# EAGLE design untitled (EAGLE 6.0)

## Sheet 1 of 3: NAP a SERVO
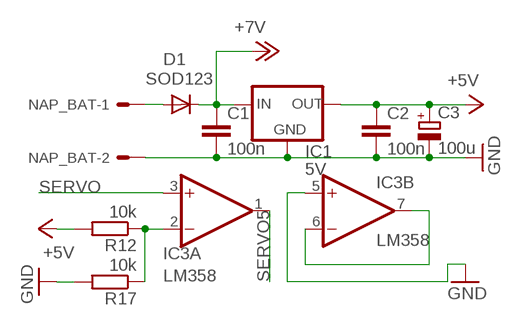
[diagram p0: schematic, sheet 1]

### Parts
C1  100n  C-EUC0805K  [C0805K]
C2  100n  C-EUC0805K  [C0805K]
C3  100u  CPOL-EUE2-5  [E2-5]
D1  SOD123  CGRM4001-G  [SOD-123_MINI-SMA]
IC1  5V  78XXL  [78XXL]
IC3  LM358  TL072D  [SO08]
NAP_BAT  22-27-2021-02  [6410-02]
R12  10k  R-EU_0207/10  [0207/10]
R17  10k  R-EU_0207/10  [0207/10]

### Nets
+7V: C1.1 D1.C IC1.IN ; also sheet 2
GND: C1.2 C2.2 C3.- IC1.GND IC3.5(B:+IN) NAP_BAT.2 R17.2 ; also sheet 2,3
N$2: D1.A NAP_BAT.1
N$6: IC3.6(B:-IN) IC3.7(B:OUT)
N$14: IC3.2(A:-IN) R12.1 R17.1
SERVO: IC3.3(A:+IN) ; also sheet 2
SERVO5: IC3.1(A:OUT) ; also sheet 2
VCC: C2.1 C3.+ IC1.OUT R12.2 ; supply symbol labelled +5V ; also sheet 2,3

## Sheet 2 of 3: HEADER_IO
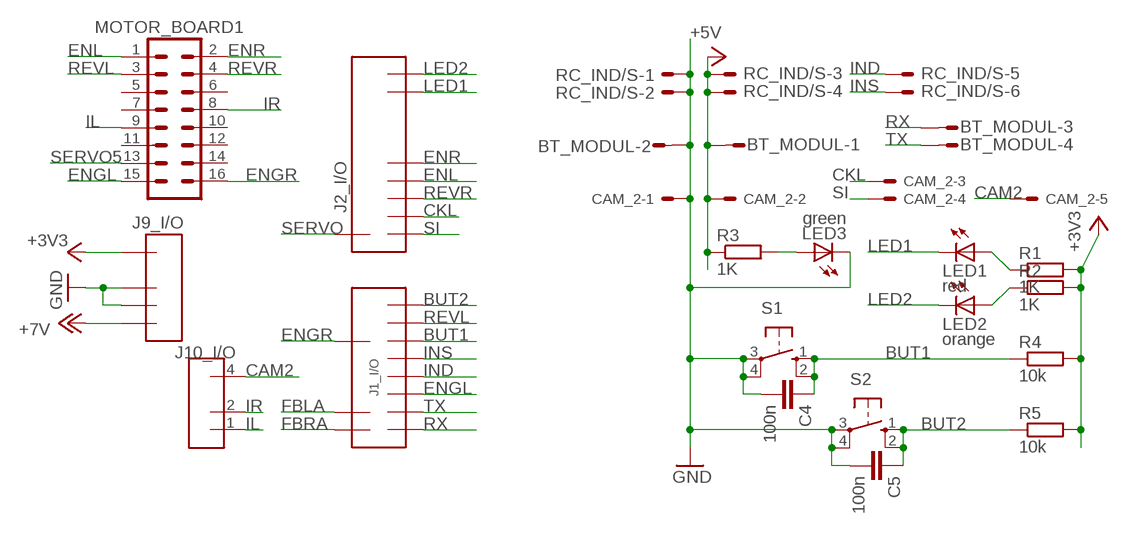
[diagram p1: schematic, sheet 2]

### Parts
BT_MODUL  M04S  [04P]
C4  100n  C-EUC0805K  [C0805K]
C5  100n  C-EUC0805K  [C0805K]
CAM_2  22-27-2051-05  [6410-05]
J1_I/O  DOLNE  [DOLNE]
J2_I/O  HORNE  [HORNE]
J9_I/O  NAP  [NAP]
J10_I/O  ANALOG  [ANALOG]
LED1  red  LED3MM  [LED3MM]
LED2  orange  LED3MM  [LED3MM]
LED3  green  LED3MM  [LED3MM]
MOTOR_BOARD1  ML16  [ML16]
R1  1K  R-EU_R0805  [R0805]
R2  1K  R-EU_R0805  [R0805]
R3  1K  R-EU_R0603  [R0603]
R4  10k  R-EU_R0805  [R0805]
R5  10k  R-EU_R0805  [R0805]
RC_IND/S  ML6E  [ML6]
S1  10-XX  [B3F-10XX]
S2  10-XX  [B3F-10XX]

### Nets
+3V3: J9_I/O.1 R1.2 R2.2 R4.2 R5.2
+7V: J9_I/O.4 ; also sheet 1
BUT1: C4.1 J1_I/O.P$9 R4.1 S1.1(S) S1.2(S1)
BUT2: C5.1 J1_I/O.P$11 R5.1 S2.1(S) S2.2(S1)
CAM2: CAM_2.5 J10_I/O.4
CKL: CAM_2.3 J2_I/O.P$3
ENGL: J1_I/O.P$5 MOTOR_BOARD1.15
ENGR: J1_I/O.P$8 MOTOR_BOARD1.16
ENL: J2_I/O.P$5 MOTOR_BOARD1.1
ENR: J2_I/O.P$6 MOTOR_BOARD1.2
FBLA: J1_I/O.P$3 ; also sheet 3
FBRA: J1_I/O.P$1 ; also sheet 3
GND: BT_MODUL.2 C4.2 C5.2 CAM_2.1 J9_I/O.2 J9_I/O.3 LED3.K(C) RC_IND/S.1 RC_IND/S.2 S1.3(P) S1.4(P1) S2.3(P) S2.4(P1) ; also sheet 1,3
IL: J10_I/O.1 MOTOR_BOARD1.9
IND: J1_I/O.P$6 RC_IND/S.5
INS: J1_I/O.P$7 RC_IND/S.6
IR: J10_I/O.2 MOTOR_BOARD1.8
LED1: J2_I/O.P$7 LED1.K(C)
LED2: J2_I/O.P$8 LED2.K(C)
N$1: LED1.A R1.1
N$15: LED2.A R2.1
N$16: LED3.A R3.2
REVL: J1_I/O.P$10 MOTOR_BOARD1.3
REVR: J2_I/O.P$4 MOTOR_BOARD1.4
RX: BT_MODUL.3 J1_I/O.P$2
SERVO: J2_I/O.P$1 ; also sheet 1
SERVO5: MOTOR_BOARD1.13 ; also sheet 1
SI: CAM_2.4 J2_I/O.P$2
TX: BT_MODUL.4 J1_I/O.P$4
VCC: BT_MODUL.1 CAM_2.2 R3.1 RC_IND/S.3 RC_IND/S.4 ; supply symbol labelled +5V ; also sheet 1,3
Unconnected: MOTOR_BOARD1.5 MOTOR_BOARD1.6 MOTOR_BOARD1.7 MOTOR_BOARD1.10 MOTOR_BOARD1.11 MOTOR_BOARD1.12 MOTOR_BOARD1.14

## Sheet 3 of 3: CNY70
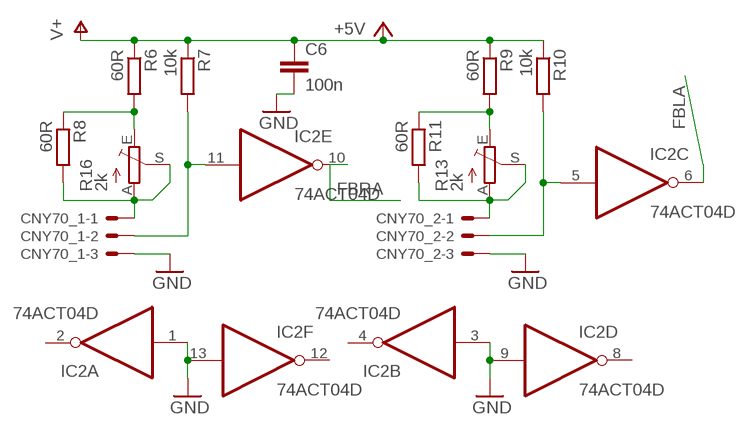
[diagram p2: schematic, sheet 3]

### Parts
C6  100n  C-EUC0805K  [C0805K]
CNY70_1  22-27-2031-03  [6410-03]
CNY70_2  22-27-2031-03  [6410-03]
IC2  74ACT04D  [SO14]
R6  60R  R-EU_R0603  [R0603]
R7  10k  R-EU_R0603  [R0603]
R8  60R  R-EU_R0603  [R0603]
R9  60R  R-EU_R0603  [R0603]
R10  10k  R-EU_R0603  [R0603]
R11  60R  R-EU_R0603  [R0603]
R13  2k  TRIM_EU-CA6V  [CA6V]
R16  2k  TRIM_EU-CA6V  [CA6V]

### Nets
FBLA: IC2.6(C:O) ; also sheet 2
FBRA: IC2.10(E:O) ; also sheet 2
GND: C6.2 CNY70_1.3 CNY70_2.3 IC2.1(A:I) IC2.3(B:I) IC2.9(D:I) IC2.13(F:I) ; also sheet 1,2
N$3: R9.2 R11.1 R13.E
N$4: R6.2 R8.1 R16.E
N$5: CNY70_2.1 R11.2 R13.A R13.S
N$8: CNY70_1.1 R8.2 R16.A R16.S
N$9: CNY70_1.2 IC2.11(E:I) R7.2
N$10: CNY70_2.2 IC2.5(C:I) R10.2
VCC: C6.1 R6.1 R7.1 R9.1 R10.1 ; supply symbol labelled V+, +5V ; also sheet 1,2
Unconnected: IC2.2(A:O) IC2.4(B:O) IC2.8(D:O) IC2.12(F:O)

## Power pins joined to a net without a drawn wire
GND: IC2.7(P:GND) IC3.4(P:V-)
VCC: IC2.14(P:VCC) IC3.8(P:V+)

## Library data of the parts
BT_MODUL = con-amp-quick:M04S: AMP QUICK CONNECTOR; OC_FARNELL: unknown; OC_NEWARK: unknown
C1 C2 C4-C6 = rcl:C-EU: CAPACITOR, European symbol
C3 = rcl:CPOL-EU: POLARIZED CAPACITOR, European symbol
CAM_2 = con-molex:22-?-05: CONNECTOR wire to board 2.54 mm (.1 inch) pitch header; OC_FARNELL: unknown; OC_NEWARK: unknown
CNY70_1 CNY70_2 = con-molex:22-?-03: CONNECTOR wire to board 2.54 mm (.1 inch) pitch header; OC_FARNELL: unknown; OC_NEWARK: unknown
D1 = diode:CGRM400*-G: Molded plasitc,JEDEC SOD-123/Mini SMA
IC1 = v-reg:78XXL: VOLTAGE REGULATOR
IC2 = 74xx-eu:74*04: Hex INVERTER
IC3 = linear:TL072: OP AMP
J1_I/O = con-tfc:DOLNE
J2_I/O = con-tfc:HORNE
J9_I/O = con-tfc:NAP
J10_I/O = con-tfc:ANALOG
LED1-LED3 = led:LED: LED
MOTOR_BOARD1 = con-ml:ML16: HARTING; OC_FARNELL: unknown; OC_NEWARK: unknown
NAP_BAT = con-molex:22-?-02: CONNECTOR; OC_FARNELL: unknown; OC_NEWARK: unknown
R1-R12 R17 = rcl:R-EU_: RESISTOR, European symbol
R13 R16 = pot:TRIM_EU-: POTENTIOMETER
RC_IND/S = con-ml:ML6E: HARTING; OC_FARNELL: unknown; OC_NEWARK: unknown
S1 S2 = switch-omron:10-XX: OMRON SWITCH; MPN: B3F-1000; OC_FARNELL: 176432; OC_NEWARK: 36M3542

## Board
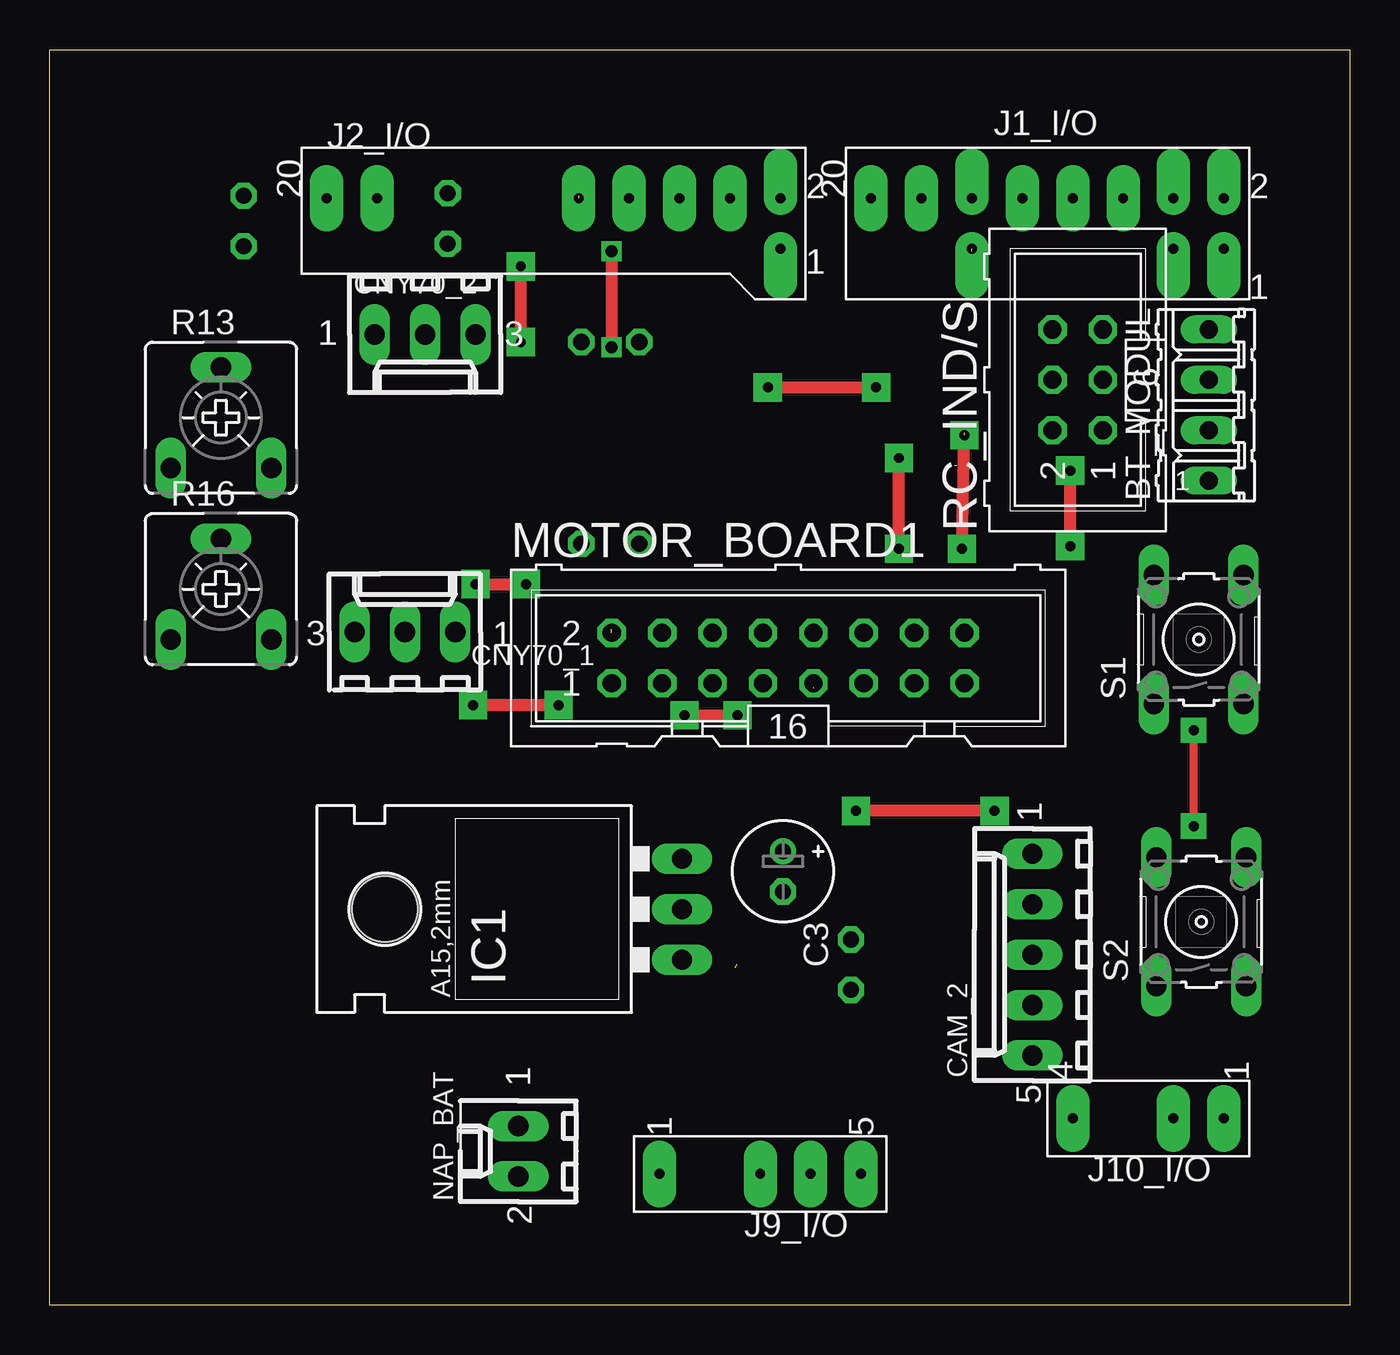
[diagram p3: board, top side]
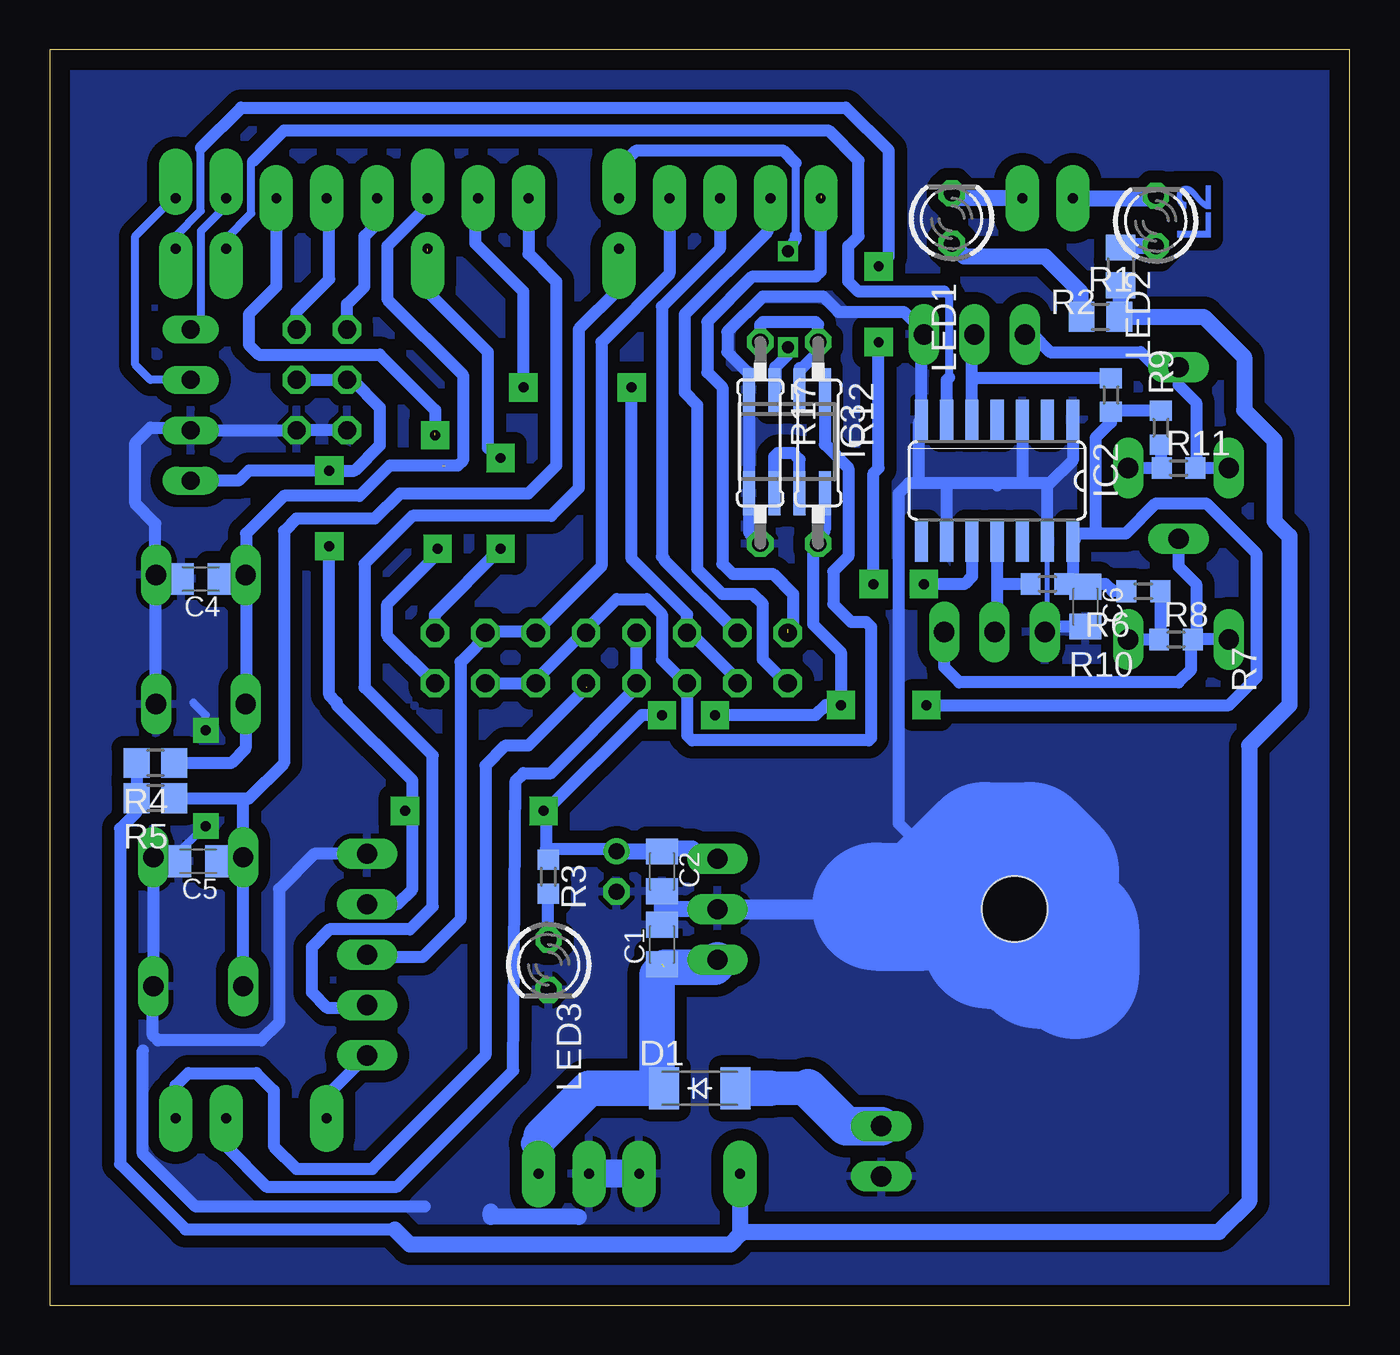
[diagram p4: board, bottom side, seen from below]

Size 65.53 x 63.25 mm. Coordinates in mm from the lower left corner, seen from the top.
Outline: 0,63.25 65.53,63.25 65.53,0 0,0 0,63.25
Copper layers (1*16): Top 0.035mm / dielectric 1.5mm / Bottom 0.035mm
Design rules: minimum track width 10mil, minimum drill 24mil, track to track 8mil, track to pad 8mil, pad to pad 8mil, via to via 8mil, smd to smd 8mil, copper to edge 40mil, drill to drill 8mil, minimum pad ring 10mil, minimum via ring 8mil, stop-mask expansion 4mil, vias tented up to drill 0mil, thermal gap 10mil

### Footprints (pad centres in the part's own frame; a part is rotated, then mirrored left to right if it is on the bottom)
04P = drill 0.914 long: 1 -3.81,0; 2 -1.27,0; 3 1.27,0; 4 3.81,0
C0805K = smd 1.3 x 1.6: 1 -1,0; 2 1,0
E2-5 = drill 0.813 pad 1.27: + -1.016,0 | drill 0.813 pad 1.27 octagon: - 1.016,0
6410-05 = drill 1.016 long: 1 5.08,0; 2 2.54,0; 3 0,0; 4 -2.54,0; 5 -5.08,0
6410-03 = drill 1.016 long: 1 2.54,0; 2 0,0; 3 -2.54,0
SOD-123_MINI-SMA = smd 1.5 x 2.1: A 1.8,0; C -1.8,0
78XXL = drill 1.016 long: GND 0,-3.81; IN -2.54,-3.81; OUT 2.54,-3.81 | hole 3.302: 0,11.176
SO14 = smd 0.66 x 2.032: 1 -3.81,-3.073; 2 -2.54,-3.073; 3 -1.27,-3.073; 4 0,-3.073; 5 1.27,-3.073; 6 2.54,-3.073; 7 3.81,-3.073; 8 3.81,3.073; 9 2.54,3.073; 10 1.27,3.073; 11 0,3.073; 12 -1.27,3.073; 13 -2.54,3.073; 14 -3.81,3.073
SO08 = smd 0.6 x 2.2: 1 -1.905,-2.6; 2 -0.635,-2.6; 3 0.635,-2.6; 4 1.905,-2.6; 5 1.905,2.6; 6 0.635,2.6; 7 -0.635,2.6; 8 -1.905,2.6
DOLNE = drill 0.5 pad 1.676 offset: P$1 8.89,-1.27; P$2 8.89,1.27; P$3 6.35,-1.27; P$4 6.35,1.27; P$8 -3.81,-1.27; P$9 -3.81,1.27 | drill 0.5 pad 1.676 long: P$5 3.81,1.27; P$6 1.27,1.27; P$7 -1.27,1.27; P$10 -6.35,1.27; P$11 -8.89,1.27
HORNE = drill 0.5 pad 1.676 offset: P$1 8.89,1.27; P$2 8.89,-1.27 | drill 0.5 pad 1.676 long: P$3 6.35,1.27; P$4 3.81,1.27; P$5 1.27,1.27; P$6 -1.27,1.27; P$7 -11.43,1.27; P$8 -13.97,1.27
NAP = drill 0.5 pad 1.676 long: 1 0,5.08; 2 0,0; 3 0,-2.54; 4 0,-5.08
ANALOG = drill 0.5 pad 1.676 long: 1 0,-3.81; 2 0,-1.27; 4 0,3.81
LED3MM = drill 0.813 octagon: A -1.27,0; K 1.27,0
ML16 = drill 0.914 octagon: 1 -8.89,-1.27; 2 -8.89,1.27; 3 -6.35,-1.27; 4 -6.35,1.27; 5 -3.81,-1.27; 6 -3.81,1.27; 7 -1.27,-1.27; 8 -1.27,1.27; 9 1.27,-1.27; 10 1.27,1.27; 11 3.81,-1.27; 12 3.81,1.27; 13 6.35,-1.27; 14 6.35,1.27; 15 8.89,-1.27; 16 8.89,1.27
6410-02 = drill 1.016 long: 1 1.27,0; 2 -1.27,0
R0805 = smd 1.3 x 1.5: 1 -0.95,0; 2 0.95,0
R0603 = smd 1 x 1.1: 1 -0.85,0; 2 0.85,0
0207/10 = drill 0.813 octagon: 1 -5.08,0; 2 5.08,0
CA6V = drill 1.016 long: A -2.54,-2.54; E 2.54,-2.54; S 0,2.54
ML6 = drill 0.914 octagon: 1 -2.54,-1.27; 2 -2.54,1.27; 3 0,-1.27; 4 0,1.27; 5 2.54,-1.27; 6 2.54,1.27
B3F-10XX = drill 1.016 long: 1 -3.251,2.261; 2 3.251,2.261; 3 -3.251,-2.261; 4 3.251,-2.261

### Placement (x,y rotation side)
BT_MODUL  58.42,45.34 90 top
C1  34.67,18.16 90 bottom
C2  34.67,21.84 270 bottom
C3  36.96,21.84 270 top
C4  57.91,36.58 180 bottom
C5  58.04,22.35 180 bottom
C6  13.33,35.18 270 bottom
CAM_2  49.53,17.65 90 top
CNY70_1  17.91,33.91 0 top
CNY70_2  18.92,48.9 180 top
D1  32.77,10.92 0 bottom
IC1  28.07,19.94 90 top
IC2  17.78,41.53 180 bottom
IC3  28.37,43.5 180 bottom
J1_I/O  50.29,54.48 0 top
J2_I/O  27.94,54.48 0 top
J9_I/O  35.81,6.6 90 top
J10_I/O  55.37,9.4 90 top
LED1  20.07,54.74 90 bottom
LED2  9.78,54.61 90 bottom
LED3  40.39,17.14 270 bottom
MOTOR_BOARD1  37.22,32.59 0 top
NAP_BAT  23.62,7.75 90 top
R1  12.57,49.78 0 bottom
R2  11.56,52.32 270 bottom
R3  40.4,21.57 270 bottom
R4  60.2,27.3 180 bottom
R5  60.2,25.53 180 bottom
R6  10.41,35.96 0 bottom
R7  15.24,36.32 180 bottom
R8  8.76,33.53 0 bottom
R9  9.53,44.2 270 bottom
R10  12.04,45.85 90 bottom
R11  8.64,42.16 0 bottom
R12  26.8,43.43 270 bottom
R13  8.64,44.7 0 top
R16  8.64,36.07 0 top
R17  29.72,43.43 270 bottom
RC_IND/S  51.82,46.61 90 top
S1  57.91,33.53 90 top
S2  58.04,19.3 90 top

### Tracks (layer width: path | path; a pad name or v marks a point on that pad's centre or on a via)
+3V3
  Bottom 0.406: 30.73,3.56 30.61,3.56 30.61,3.68
  Bottom 0.61: R4.2 R5.2 61.15,24.83 61.98,24 61.98,7.11 58.67,3.81 48.13,3.81 | 30.61,6.48 J9_I/O.1
  Bottom 0.813: R2.2 11.56,49.85 R1.2 7.37,49.78 5.33,47.75 5.33,45.09 3.81,43.56 3.81,39.5 3.05,38.73 3.05,30.23 5.08,28.19 5.08,5.21 6.6,3.68 30.61,3.68 | J9_I/O.1 30.73,3.56 31.24,3.05 47.37,3.05 48.13,3.81
+7V  (1 unrouted)
  Bottom 0.406: J9_I/O.4 41.02,6.6 41.02,8.25 | D1.C 34.93,10.92
  Bottom 1.27: 40.77,8.51 41.02,8.25 41.15,8.13
  Bottom 1.778: IC1.IN 31.88,17.14 32,17.02 34.54,17.02 34.93,16.64 34.93,10.92 38.35,10.92 40.77,8.51
BUT1  (1 unrouted)
  Bottom 0.406: C4.1 55.75,36.58 55.63,36.7
  Bottom 0.61: J1_I/O.P$9 46.48,55.37 48.51,53.34 48.51,50.67 44.7,46.86 44.7,42.55 44.96,42.29 45.59,42.29 | R4.1 56.39,27.3 55.65,28.04 S1.1 55.63,30.3 55.63,36.58 55.75,36.58 55.75,36.68 S1.2 55.63,36.8 55.63,38.86 53.72,40.77 49.91,40.77 48.39,42.29 45.72,42.29
BUT2
  Bottom 0.61: J1_I/O.P$11 41.4,52.96 40.01,51.56 40.01,42.29 41.4,40.89 47.88,40.89 49.15,39.62 53.09,39.62 53.72,38.99 53.72,27.3 55.5,25.53 55.75,25.53 | C5.1 55.98,22.35 S2.2 | S2.2 S2.1 55.75,16.08 | R5.1 55.75,25.53 | S2.2 55.78,25.5 55.75,25.53
CAM2
  Bottom 0.61: J10_I/O.4 51.56,10.54 CAM_2.5
CKL
  Bottom 0.61: J2_I/O.P$3 34.29,51.94 37.72,48.51 37.72,37.21 41.02,33.91 43.31,33.91 44.83,32.39 44.83,19.43 46.74,17.53 49.4,17.53 CAM_2.3
ENGL  (via drill 0.5 pad 1.42)  (1 unrouted)
  Top 0.61: v45.97,38.1 v46.1,43.81
  Bottom 0.61: J1_I/O.P$5 54.1,51.31 55.5,49.91 55.5,48.39 54.99,47.88 48.9,47.88 46.1,45.09 46.1,43.94 | MOTOR_BOARD1.15 48.51,33.72 48.51,35.31 45.97,37.85 v45.97,38.1
ENGR  (via drill 0.5 pad 1.42)  (1 unrouted)
  Top 0.61: v42.8,38.1 v42.8,42.67
  Bottom 0.61: MOTOR_BOARD1.16 46.11,34.79 v42.8,38.1 | 46.48,51.05 46.48,51.44 | 46.48,51.44 46.48,53.09 46.36,53.21 | v42.8,42.67 42.93,42.67 43.43,43.18 43.43,48.01 46.36,50.93 46.36,51.31 46.48,51.44
ENL
  Bottom 0.61: MOTOR_BOARD1.1 28.4,31.32 29.59,32.51 29.59,35.31 30.1,35.81 31.62,35.81 32.89,37.08 32.89,45.34 33.53,45.97 33.53,49.91 29.34,54.1 29.34,55.63 J2_I/O.P$5
ENR  (2 unrouted)
  Bottom 0.61: 28.32,34.04 28.07,34.29 28.07,35.81 29.08,36.83 31.12,36.83 31.62,37.34 31.62,46.23 32.38,46.99 32.38,49.53 30.1,51.82 26.92,51.82 26.67,52.07 26.67,55.88
FBLA
  Bottom 0.406: 20.19,46.74 20.19,50.8 20.45,51.05 | 56.64,53.34 56.64,53.72 55.37,54.99 55.37,57.66 | 55.37,57.66 55.25,57.78 | 55.37,57.66 55.25,57.66
  Bottom 0.61: IC2.6 20.32,46.61 20.19,46.74 | 20.45,51.05 24.77,51.05 25.27,51.56 25.27,53.34 24.77,53.85 24.77,57.66 26.29,59.18 53.72,59.18 55.25,57.66 | J1_I/O.P$3 56.64,53.34
FBRA  (via drill 0.5 pad 1.42)
  Top 0.61: v21.46,36.32 v24,36.32 | v23.75,48.51 v23.75,52.32
  Bottom 0.406: J1_I/O.P$1 59.18,53.85 57.91,55.12 57.91,58.29
  Bottom 0.61: IC2.10 19.05,36.7 19.43,36.32 v21.46,36.32 | v24,36.32 24,41.91 23.75,42.16 v23.75,48.51 | v23.75,52.32 23.24,52.83 23.24,58.17 25.4,60.33 55.88,60.33 57.91,58.29
GND  (via drill 0.5 pad 1.27)
  Top 0.406: v57.66,24.13 v57.66,28.96
  Bottom 0.254: CNY70_1.3 15.24,34.04 IC2.13 | 59.36,22.55 59.24,22.55
  Bottom 0.406: C4.2 59.97,36.58 S1.4 | 17.27,18.16 16.51,18.16 16.51,20.95 15.11,20.95 | S2.4 59.36,22.55 v57.66,24.13 | v57.66,28.96 57.66,29.72 58.29,30.35
  Bottom 0.61: IC2.1 13.97,42.55 15.11,41.4 15.37,41.4 | 15.37,41.4 16.64,41.4 | 16.64,41.4 17.65,41.4 | 17.65,41.4 20.45,41.4 | 21.72,41.4 21.72,44.48 IC2.7 21.59,48.77 CNY70_2.3 21.59,49.02 | IC2.13 15.24,41.27 15.37,41.4 | 17.78,41.27 17.65,41.4 | 16.64,41.4 16.51,41.53 IC2.3 | IC2.9 20.32,41.27 20.45,41.4 | R17.2 30.28,38.91 IC3.5 IC3.4 30.28,46.91 31.37,48.01 31.37,49.02 29.59,50.8 26.54,50.8 25.78,50.04 22.48,50.04 21.46,49.02 | 20.45,41.4 21.72,41.4 | 21.72,41.4 22.23,41.4 22.73,40.89 22.73,24.26 21.59,23.11 16.13,23.11 | C6.2 15.22,34.18 15.37,34.04 | RC_IND/S.2 RC_IND/S.1 BT_MODUL.2 | S1.4 60.43,36.98 60.43,37.24 60.2,37.47 60.2,39.37 61.21,40.39 61.21,43.43 60.45,44.2 58.42,44.2 | S2.4 60.3,17.02 | 60.3,17.02 S2.3 | S2.3 60.3,16.03 60.33,16 | 60.43,17.14 60.3,17.02 | 59.24,22.55 C5.2 | 59.97,36.58 60.07,36.58 60.2,36.45 60.2,30.3 S1.3 | CAM_2.1 52.2,22.73 53.98,20.95 53.98,14.22 54.86,13.34 60.07,13.34 60.33,13.59 60.33,16.03 S2.3 | LED3.K 40.01,15.88 | 34.78,19.05 C1.2 | 46.61,4.95 58.17,4.95 60.83,7.62 60.83,12.83
  Bottom 0.813: IC1.GND 34.67,19.94 | 34.67,19.94 C2.2 34.69,20.83 | 34.67,19.94 C1.2 | 38.86,4.45 43.31,4.45 43.31,4.7
  Bottom 1.016: IC1.GND 24.64,19.94 24,19.94 23.88,20.07
  Bottom 1.422: J9_I/O.2 J9_I/O.3 | 24.77,19.81 24.64,19.94
  Bottom 6.452: 23.88,20.07 21.46,20.07 18.42,23.11 16.13,23.11 14.86,21.84 14.86,21.59 18.29,18.16 17.27,18.16 16.76,18.16 15.75,17.14 15.62,17.14 13.84,18.92 13.84,16.64
  pour Bottom (isolate 0.61): -0.38,63.37 65.79,63.37 65.79,-0.38 -0.38,-0.38
IL  (1 unrouted)
  Bottom 0.61: MOTOR_BOARD1.9 38.49,31.1 | J10_I/O.1 59.18,11.05 58.55,11.68 55.12,11.68 54.23,10.79 54.23,8 53.09,6.86 49.28,6.86 43.56,12.57 43.56,27.18 42.55,28.19 41.4,28.19 38.48,31.11
IND
  Bottom 0.61: RC_IND/S.5 53.09,50.04 51.44,51.69 51.44,55.63 J1_I/O.P$6
INS
  Bottom 0.61: RC_IND/S.6 50.55,50.42 49.66,51.31 49.66,53.85 49.15,54.36 49.15,55.63 J1_I/O.P$7
IR
  Bottom 0.61: MOTOR_BOARD1.8 35.94,33.85 35.94,31.11 40.26,26.8 41.66,26.8 42.04,26.42 42.16,11.81 48.01,5.97 54.61,5.97 56.64,8 J10_I/O.2
LED1
  Bottom 0.813: J2_I/O.P$7 19.81,55.75 LED1.K
LED2
  Bottom 0.813: J2_I/O.P$8 9.91,55.75 LED2.K
N$1
  Bottom 0.813: LED1.A 19.43,52.83 15.37,52.83 13.59,51.05 13.59,49.85 R1.1
N$2
  Bottom 0.406: 30.73,10.92 D1.A
  Bottom 1.676: 27.3,10.92 29.21,10.92
  Bottom 1.778: 29.21,10.92 30.73,10.92
  Bottom 1.93: NAP_BAT.1 25.4,9.02 27.3,10.92
N$3
  Bottom 0.61: R13.E R11.1 9.53,42.2 R9.2
N$4
  Bottom 0.61: R16.E R8.1 9.56,33.58 R6.2
N$5
  Bottom 0.61: CNY70_2.1 16,48.9 15.11,48.01 10.54,48.01 9.78,47.24 R13.S 8.64,46.35 7.75,45.47 7.75,42.2 R11.2 R13.A
N$6
  Bottom 0.61: IC3.7 27.74,42.59 28.07,42.93 28.83,42.93 29.01,42.75 IC3.6
N$7
  pour Bottom (isolate 0.61): -0.38,63.37 65.79,63.37 65.79,-0.38 -0.38,-0.38
N$8
  Bottom 0.61: R16.A R8.2 | R16.S 8.64,37.21 7.75,36.32 7.75,33.69 R8.2 | R8.2 8,33.44 8,32 8.64,31.37 19.69,31.37 20.45,32.13 CNY70_1.1
N$9
  Bottom 0.61: IC2.11 17.78,36.32 | 17.78,36.32 17.78,34.04 CNY70_1.2 | R7.2 17.78,36.32
N$10
  Bottom 0.61: IC2.5 19.05,46.48 | 19.05,46.48 19.05,48.77 CNY70_2.2 | R10.2 18.84,46.7 19.05,46.48
N$14
  Bottom 0.61: IC3.2 27.74,47.19 27.61,47.19 26.8,48.01 R12.1 26.8,49.4 26.92,49.53 29.59,49.53 29.72,49.4 R17.1
N$15
  Bottom 0.813: LED2.A 11.49,53.34 R2.1
N$16
  Bottom 0.61: LED3.A 40.4,18.41 R3.2
REVL  (via drill 0.5 pad 1.42)
  Top 0.61: v36.2,46.23 v41.66,46.23
  Bottom 0.61: MOTOR_BOARD1.3 30.87,31.51 33.4,34.04 33.4,34.8 36.2,37.59 v36.2,46.23 | v41.66,46.23 41.66,51.05 44.07,53.47 44.07,55.63 J1_I/O.P$10
REVR
  Bottom 0.61: J2_I/O.P$4 31.75,53.21 34.67,50.29 34.67,37.72 34.54,37.59 34.54,37.53 MOTOR_BOARD1.4
RX
  Bottom 0.406: BT_MODUL.3 60.45,46.61 61.21,47.37 61.21,53.85 59.31,55.75 J1_I/O.P$2
SERVO  (via drill 0.6)
  Top 0.61: v28.32,53.09 v28.32,48.26
  Bottom 0.406: 27.94,57.53 27.94,53.85
  Bottom 0.61: J2_I/O.P$1 36.83,57.28 35.94,58.17 28.58,58.17 27.94,57.53 | 27.94,53.85 27.94,53.72 v28.32,53.09 | v28.32,48.26 28.32,47.88 28.96,47.24 28.96,46.15 IC3.3
SERVO5
  Bottom 0.61: MOTOR_BOARD1.13 41.2,31.32 36.96,35.56 35.43,35.56 34.67,34.8 34.67,32.51 33.4,31.24 33.4,28.7 33.15,28.45 24.26,28.45 24.13,28.57 24.13,34.16 24.38,34.42 25.15,34.42 26.04,35.31 26.04,36.96 25.27,37.72 25.27,42.16 26.47,43.36 IC3.1
SI
  Bottom 0.61: J2_I/O.P$2 36.83,51.18 38.86,49.15 38.86,41.15 40.26,39.75 47.24,39.75 49.66,37.34 49.66,31.11 46.23,27.69 46.23,20.07 47.37,18.92 51.44,18.92 52.32,18.03 52.32,15.75 51.56,14.99 49.66,14.99 CAM_2.4
TX
  Bottom 0.406: J1_I/O.P$4 56.64,55.37 57.91,54.1 57.91,49.66 BT_MODUL.4
VCC  (via drill 0.5 pad 1.42)
  Top 0.61: v51.44,38.23 v51.44,42.04 | v47.62,24.89 v40.64,24.89 | v25.65,30.23 v21.34,30.23 | v32,29.72 v34.67,29.72
  Bottom 0.61: C3.+ 37.08,22.99 40.39,22.99 | R9.1 11.99,45.05 R10.1 12.04,44.47 12.83,43.69 12.83,39.12 12.57,38.86 | 12.57,38.86 11.3,38.86 9.78,40.39 7.24,40.39 4.7,37.85 4.7,31.62 6.1,30.23 v21.34,30.23 | 12.57,38.86 13.84,38.86 13.84,38.58 IC2.14 13.97,36.74 R7.1 | R6.1 11.95,35.96 12.32,36.32 13.59,36.32 13.84,36.07 14.1,36.32 R7.1 | C6.1 14.25,36.18 R7.1 | IC3.8 26.47,39.07 R12.2 26.8,38.1 27.05,37.85 27.05,34.29 25.65,32.89 v25.65,30.23 26.42,30.23 26.92,29.72 v32,29.72 | RC_IND/S.3 RC_IND/S.4 50.29,46.61 48.9,45.21 48.9,43.31 50.16,42.04 v51.44,42.04 55.5,42.04 56.01,41.53 BT_MODUL.1 | CAM_2.2 48.01,20.19 47.24,20.95 47.24,24.89 | 47.24,24.89 47.24,26.42 51.05,30.23 51.05,30.35 51.44,30.73 v51.44,38.23 | 47.24,24.89 v47.62,24.89 | v40.64,24.89 40.51,24.89 | 40.51,24.89 40.51,22.99 40.39,22.99 | R3.1 40.39,22.43 40.39,22.99 | v34.67,29.72 35.69,29.72 40.51,24.89
  Bottom 0.813: IC1.OUT 32.64,22.48 33.15,22.99 34.53,22.99 C2.1 36.94,22.84 C3.+

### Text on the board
Bottom: L2 | 2015 | CAM | BAT | AROS v1.1 | BU2 | BU1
